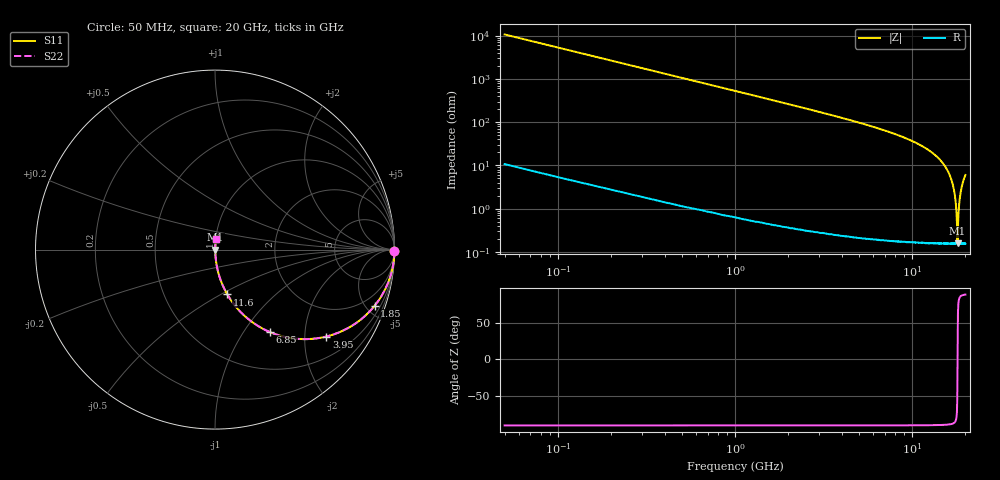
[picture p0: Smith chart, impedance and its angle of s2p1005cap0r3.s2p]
!	AVX	Thin	Film	Operation
!	Date:	March 2012
!	Description: Ultra-Miniature 01005 Size ACCU - P® Thin Film RF / Microwave Capacitor
!	Part Number:  C005YJ0R3ABSTR
!	Serial	Measurements
#	MHz	S	db	R	50
!	S11	S21	S12	S22
!	dB	Phase	dB	Phase	dB	Phase	dB	Phase
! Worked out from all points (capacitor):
!   400 points, 50 MHz to 20 GHz, reference 50 ohm
!   read as one part in series: C = 300 fF near 150 MHz
!   lowest |Z| = 160 mohm at 18.05 GHz (marker M1)
!   series resonance near 18.06 GHz, so ESL is about 260 pH
!   S11 on the Smith chart (normalised r, x): 50 MHz: open; 1.85 GHz: 1.01, -5.68; 3.95 GHz: 1.00, -2.56; 6.85 GHz: 1.00, -1.33; 11.6 GHz: 1.00, -0.54; 20 GHz: 1.00, +0.12
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50  -0.00 -0.5  -40.52 89.4  -40.52 89.4  -0.00 -0.5
100  -0.00 -1.1  -34.49 88.9  -34.49 88.9  -0.00 -1.1
200  -0.01 -2.2  -28.48 87.8  -28.48 87.8  -0.01 -2.2
500  -0.04 -5.4  -20.55 84.5  -20.55 84.5  -0.04 -5.4
1050  -0.17 -11.2  -14.21 78.7  -14.21 78.7  -0.17 -11.2
1850  -0.51 -19.4  -9.57 70.5  -9.57 70.5  -0.51 -19.4
3400  -1.59 -33.6  -5.15 56.3  -5.15 56.3  -1.59 -33.6
3950  -2.08 -38.0  -4.22 51.9  -4.22 51.9  -2.08 -38.0
6700  -4.99 -55.6  -1.67 34.3  -1.67 34.3  -4.99 -55.6
6850  -5.16 -56.3  -1.59 33.5  -1.59 33.5  -5.16 -56.3
10050  -9.32 -69.8  -0.55 20.0  -0.55 20.0  -9.32 -69.8
11600  -11.73 -74.6  -0.32 15.0  -0.32 15.0  -11.73 -74.6
13350  -15.04 -79.3  -0.15 10.2  -0.15 10.2  -15.04 -79.3
15350  -20.42 -83.6  -0.05 5.5  -0.05 5.5  -20.42 -83.6
16700  -26.78 -85.4  -0.02 2.6  -0.02 2.6  -26.78 -85.4
17650  -37.45 -82.5  -0.01 0.8  -0.01 0.8  -37.45 -82.5
17900  -45.50 -72.6  -0.01 0.3  -0.01 0.3  -45.50 -72.6
18050  -56.05 -6.5  -0.01 0.0  -0.01 0.0  -56.05 -6.5
18250  -43.77 75.7  -0.01 -0.4  -0.01 -0.4  -43.77 75.7
18600  -35.14 83.9  -0.01 -1.0  -0.01 -1.0  -35.14 83.9
19150  -29.23 85.4  -0.02 -2.0  -0.02 -2.0  -29.23 85.4
20000  -24.43 85.1  -0.03 -3.4  -0.03 -3.4  -24.43 85.1
